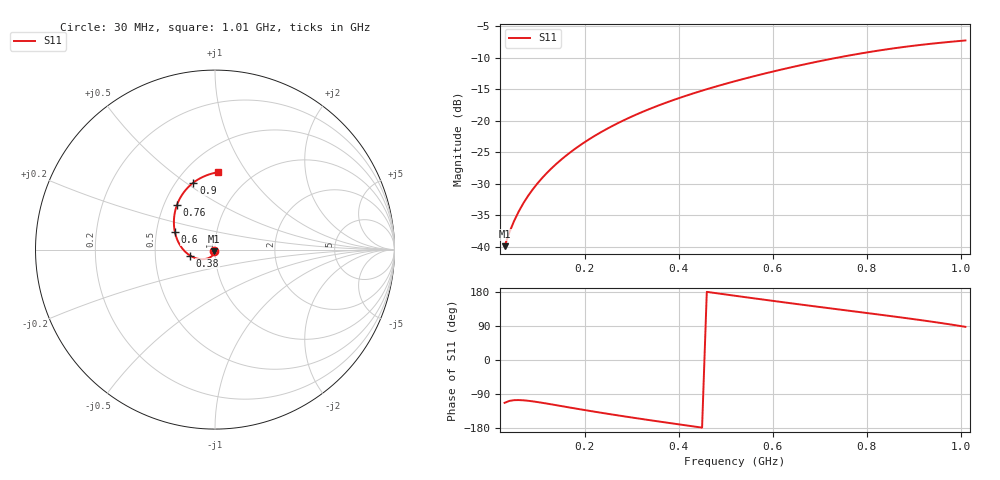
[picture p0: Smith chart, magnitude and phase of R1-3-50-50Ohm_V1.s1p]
!version-1
!date-08.2020
!Series
#	GHZ S RI R 50.0
!	FREQ.GHZ	S11RE	S11IM
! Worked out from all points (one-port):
!   99 points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, 30 MHz to 1.01 GHz, reference 50 ohm
!   lowest |S11| = -39.9 dB at 30 MHz (marker M1), VSWR 1.02, Z = 49.6 - j0.926 ohm
!   |S11| at or under -10 dB: start of sweep to 739.3 MHz
!   S11 on the Smith chart (normalised r, x): 30 MHz: 0.99, -0.02; 380 MHz: 0.76, -0.05; 600 MHz: 0.62, +0.13; 760 MHz: 0.58, +0.33; 900 MHz: 0.61, +0.54; 1.01 GHz: 0.71, +0.75
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0.03  -0.00397 -0.00933
0.04  -0.00401 -0.0124
0.05  -0.00441 -0.0154
0.06  -0.00517 -0.0184
0.07  -0.00626 -0.0213
0.08  -0.00768 -0.0242
0.1  -0.0114 -0.0298
0.12  -0.0163 -0.035
0.14  -0.0222 -0.0397
0.16  -0.0291 -0.0438
0.19  -0.0409 -0.0488
0.22  -0.0542 -0.0521
0.28  -0.0841 -0.0528
0.33  -0.1108 -0.0466
0.38  -0.1377 -0.0339
0.4  -0.1481 -0.0269
0.46  -0.1775 0.000577
0.52  -0.202 0.0373
0.6  -0.2237 0.099
0.65  -0.2289 0.1433
0.71  -0.2249 0.2002
0.76  -0.2118 0.2489
0.77  -0.208 0.2586
0.83  -0.1767 0.3151
0.89  -0.1294 0.3658
0.9  -0.1199 0.3734
0.96  -0.0521 0.4117
1.01  0.0188 0.4314
